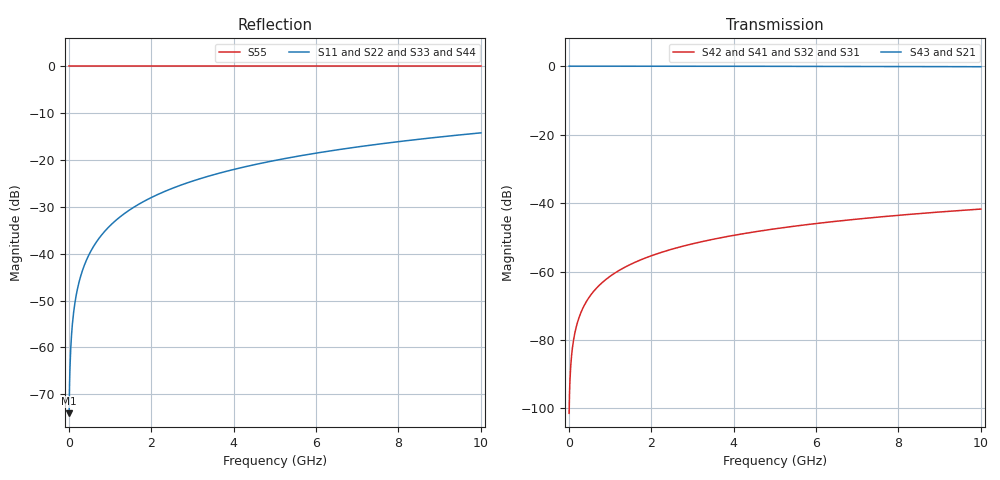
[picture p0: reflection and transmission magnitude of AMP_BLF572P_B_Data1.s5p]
! Created Mon Jul 19 16:16:05 2010
# ghz S ma R 50
! 5 Port Network Data from SP1.SP block
! freq  magS11  angS11  magS12  angS12  magS13  angS13  magS14  angS14
!  magS15  angS15
!  magS21  angS21  magS22  angS22  magS23  angS23
!  magS24  angS24  magS25  angS25
!  magS31  angS31  magS32  angS32
!  magS33  angS33  magS34  angS34  magS35  angS35
!  magS41  angS41
!  magS42  angS42  magS43  angS43  magS44  angS44  magS45  angS45
!  magS51  angS51  magS52  angS52  magS53  angS53  magS54  angS54
!  magS55  angS55
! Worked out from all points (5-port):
!   1000 points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, 10 MHz to 10 GHz, reference 50 ohm
!   strongest paths, dB at 10 MHz, 2.51 GHz, 5.01 GHz, 7.51 GHz, 10 GHz:
!     S43: 0.0, 0.0, 0.0, -0.1, -0.2
!     S21: 0.0, 0.0, 0.0, -0.1, -0.2
!     S42: -101.4, -53.4, -47.5, -44.1, -41.7
!     S41: -101.4, -53.4, -47.5, -44.1, -41.7
!     S32: -101.4, -53.4, -47.5, -44.1, -41.7
!     S31: -101.4, -53.4, -47.5, -44.1, -41.7
!   lowest |S11| = -74.1 dB at 10 MHz (marker M1), VSWR 1.00, Z = 50 + j0.0198 ohm
!   |S11| at or under -10 dB: start of sweep to end of sweep
